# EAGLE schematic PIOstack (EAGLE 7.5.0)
COPYRIGHT: © 2015/2016 luani.de; LICENSE: CC-BY-SA 4.0; PROJEKT: PIOstack – Raspb. Pi Zero LAN, USB & Audio; REVISION: 1.1
Assembly variants: 2-Port Hub Minimal

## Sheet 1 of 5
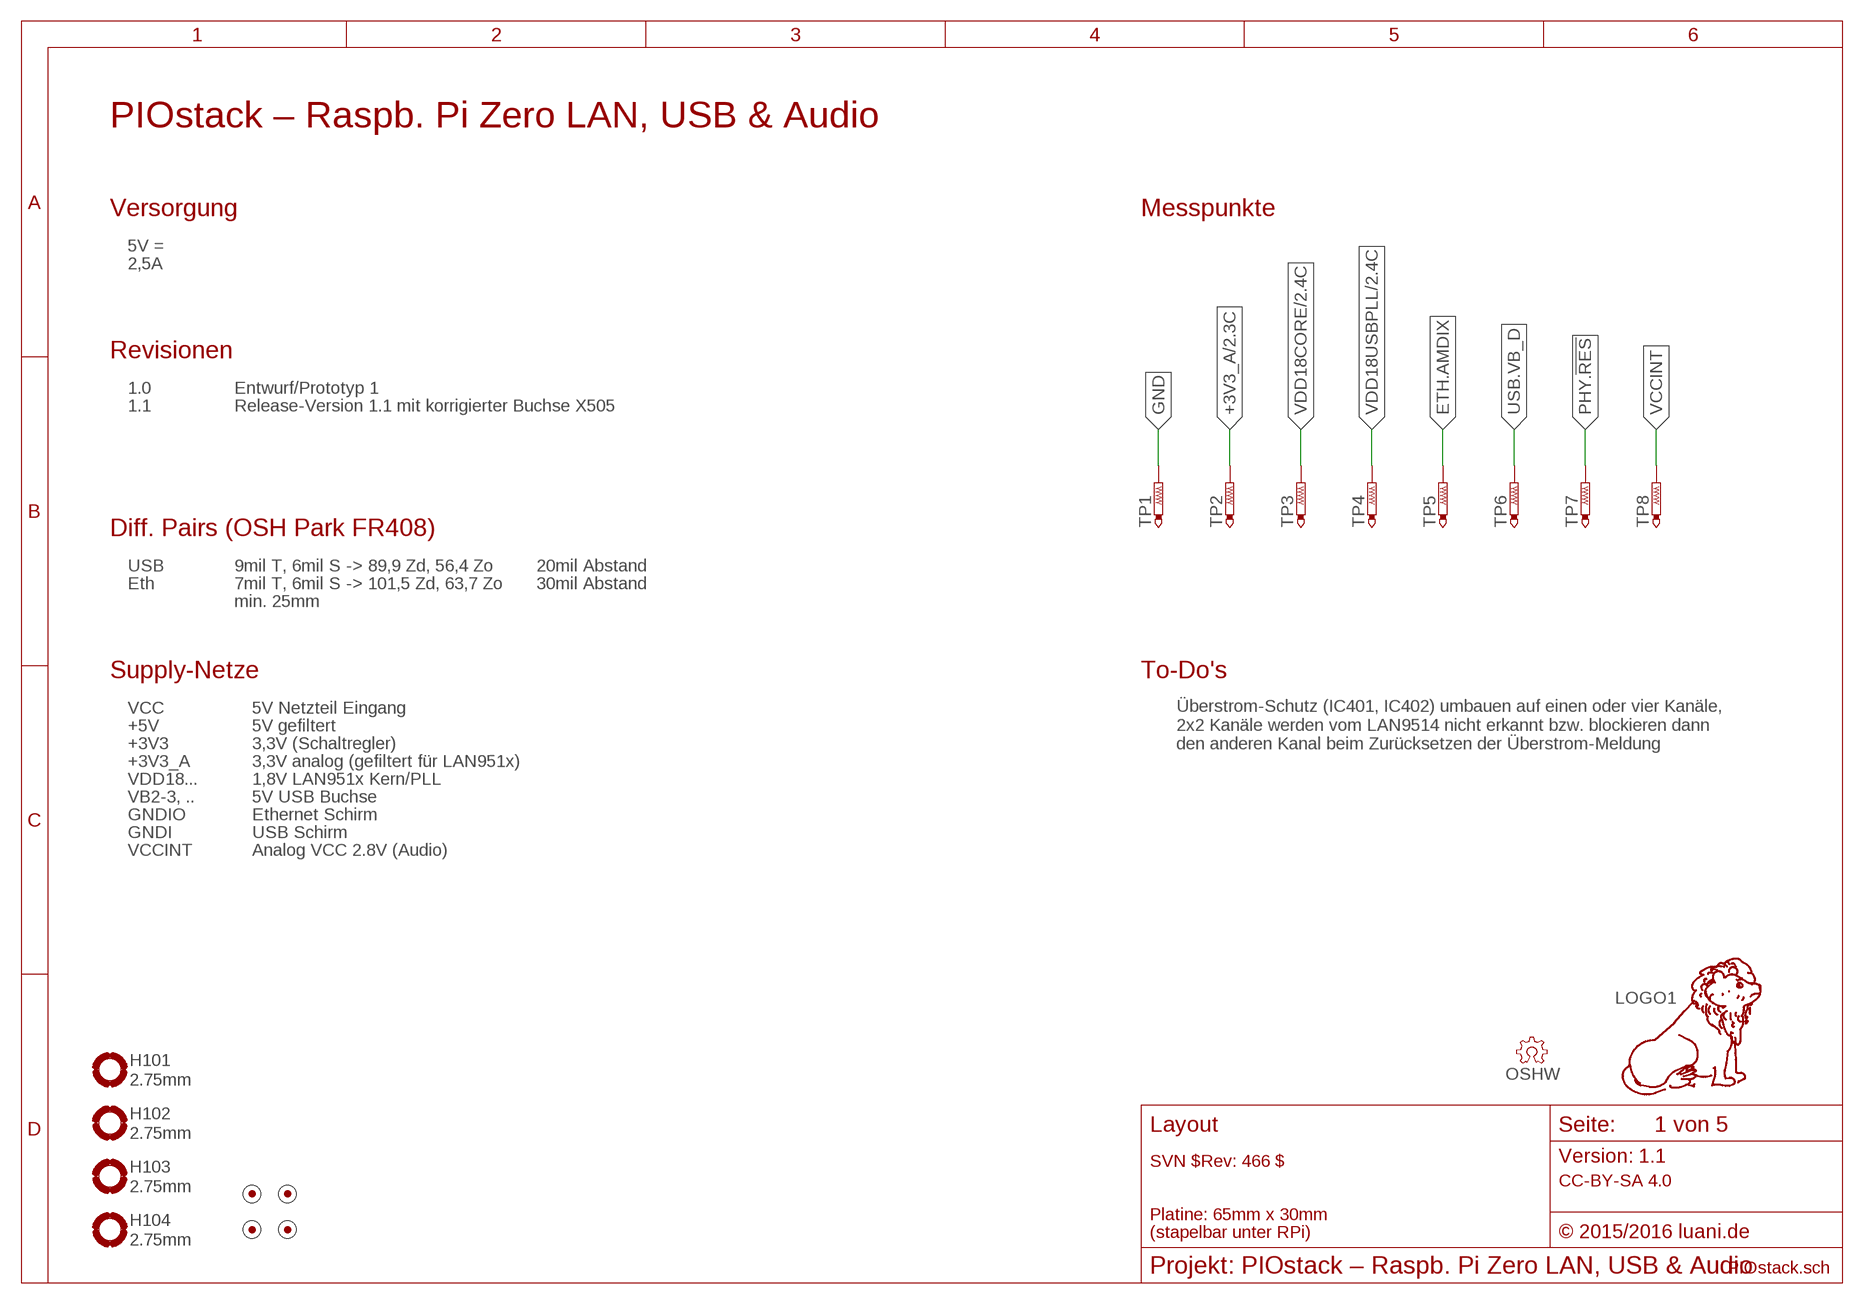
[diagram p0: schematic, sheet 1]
FRAME101 (FRAME_A4-L): TEXT-1: Layout; TEXT-2: SVN $Rev: 466 $; TEXT-4: Platine: 65mm x 30mm; TEXT-5: (stapelbar unter RPi)

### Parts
H101  2.75mm  HOLE_2.75R  [HOLE_2.75R]
H102  2.75mm  HOLE_2.75R  [HOLE_2.75R]
H103  2.75mm  HOLE_2.75R  [HOLE_2.75R]
H104  2.75mm  HOLE_2.75R  [HOLE_2.75R]
LOGO1  LOGO-10MM-TPLACE  [10MM-TPLACE]
MARK101  FIDUCIAL-1.0/CREAM  [FIDUCIAL-1MM/CREAM]
MARK102  FIDUCIAL-1.0/CREAM  [FIDUCIAL-1MM/CREAM]
MARK103  FIDUCIAL-1.0/CREAM  [FIDUCIAL-1MM/CREAM]
MARK104  FIDUCIAL-1.0/CREAM  [FIDUCIAL-1MM/CREAM]
OSHW  OSHW-3MM-FILL-TPLACE  [OSHW-FILL-3MM-TPLACE]
TP1  PTR1TP07R  [TP07R]
TP2  PTR1TP07R  [TP07R]
TP3  PTR1TP07R  [TP07R]
TP4  PTR1TP07R  [TP07R]
TP5  PTR1TP07R  [TP07R]
TP6  PTR1TP07R  [TP07R]
TP7  PTR1TP07R  [TP07R]
TP8  PTR1TP07R  [TP07R]

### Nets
+3V3_A: TP2.TP ; also sheet 2,3
ETH.AMDIX: TP5.TP ; also sheet 3
GND: TP1.TP ; also sheet 2,3,4,5
PHY.!RES: TP7.TP ; also sheet 2
USB.VB_D: TP6.TP ; also sheet 4
VCCINT: TP8.TP ; also sheet 5
VDD18CORE: TP3.TP ; also sheet 2
VDD18USBPLL: TP4.TP ; also sheet 2

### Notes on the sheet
- Versorgung | Messpunkte
- 5V =
- 2,5A
- Revisionen
- 1.0 | Entwurf/Prototyp 1
- 1.1 | Release-Version 1.1 mit korrigierter Buchse X505
- Diff. Pairs (OSH Park FR408)
- USB | 9mil T, 6mil S -> 89,9 Zd, 56,4 Zo | 20mil Abstand
- Eth | 7mil T, 6mil S -> 101,5 Zd, 63,7 Zo | 30mil Abstand
- min. 25mm
- Supply-Netze | To-Do's
- VCC | 5V Netzteil Eingang
- +5V | 5V gefiltert
- +3V3 | 3,3V (Schaltregler)
- Überstrom-Schutz (IC401, IC402) umbauen auf einen oder vier Kanäle,
  2x2 Kanäle werden vom LAN9514 nicht erkannt bzw. blockieren dann
  den anderen Kanal beim Zurücksetzen der Überstrom-Meldung
- +3V3_A | 3,3V analog (gefiltert für LAN951x)
- VDD18... | 1,8V LAN951x Kern/PLL
- VB2-3, .. | 5V USB Buchse
- GNDIO | Ethernet Schirm
- GNDI | USB Schirm
- VCCINT | Analog VCC 2.8V (Audio)

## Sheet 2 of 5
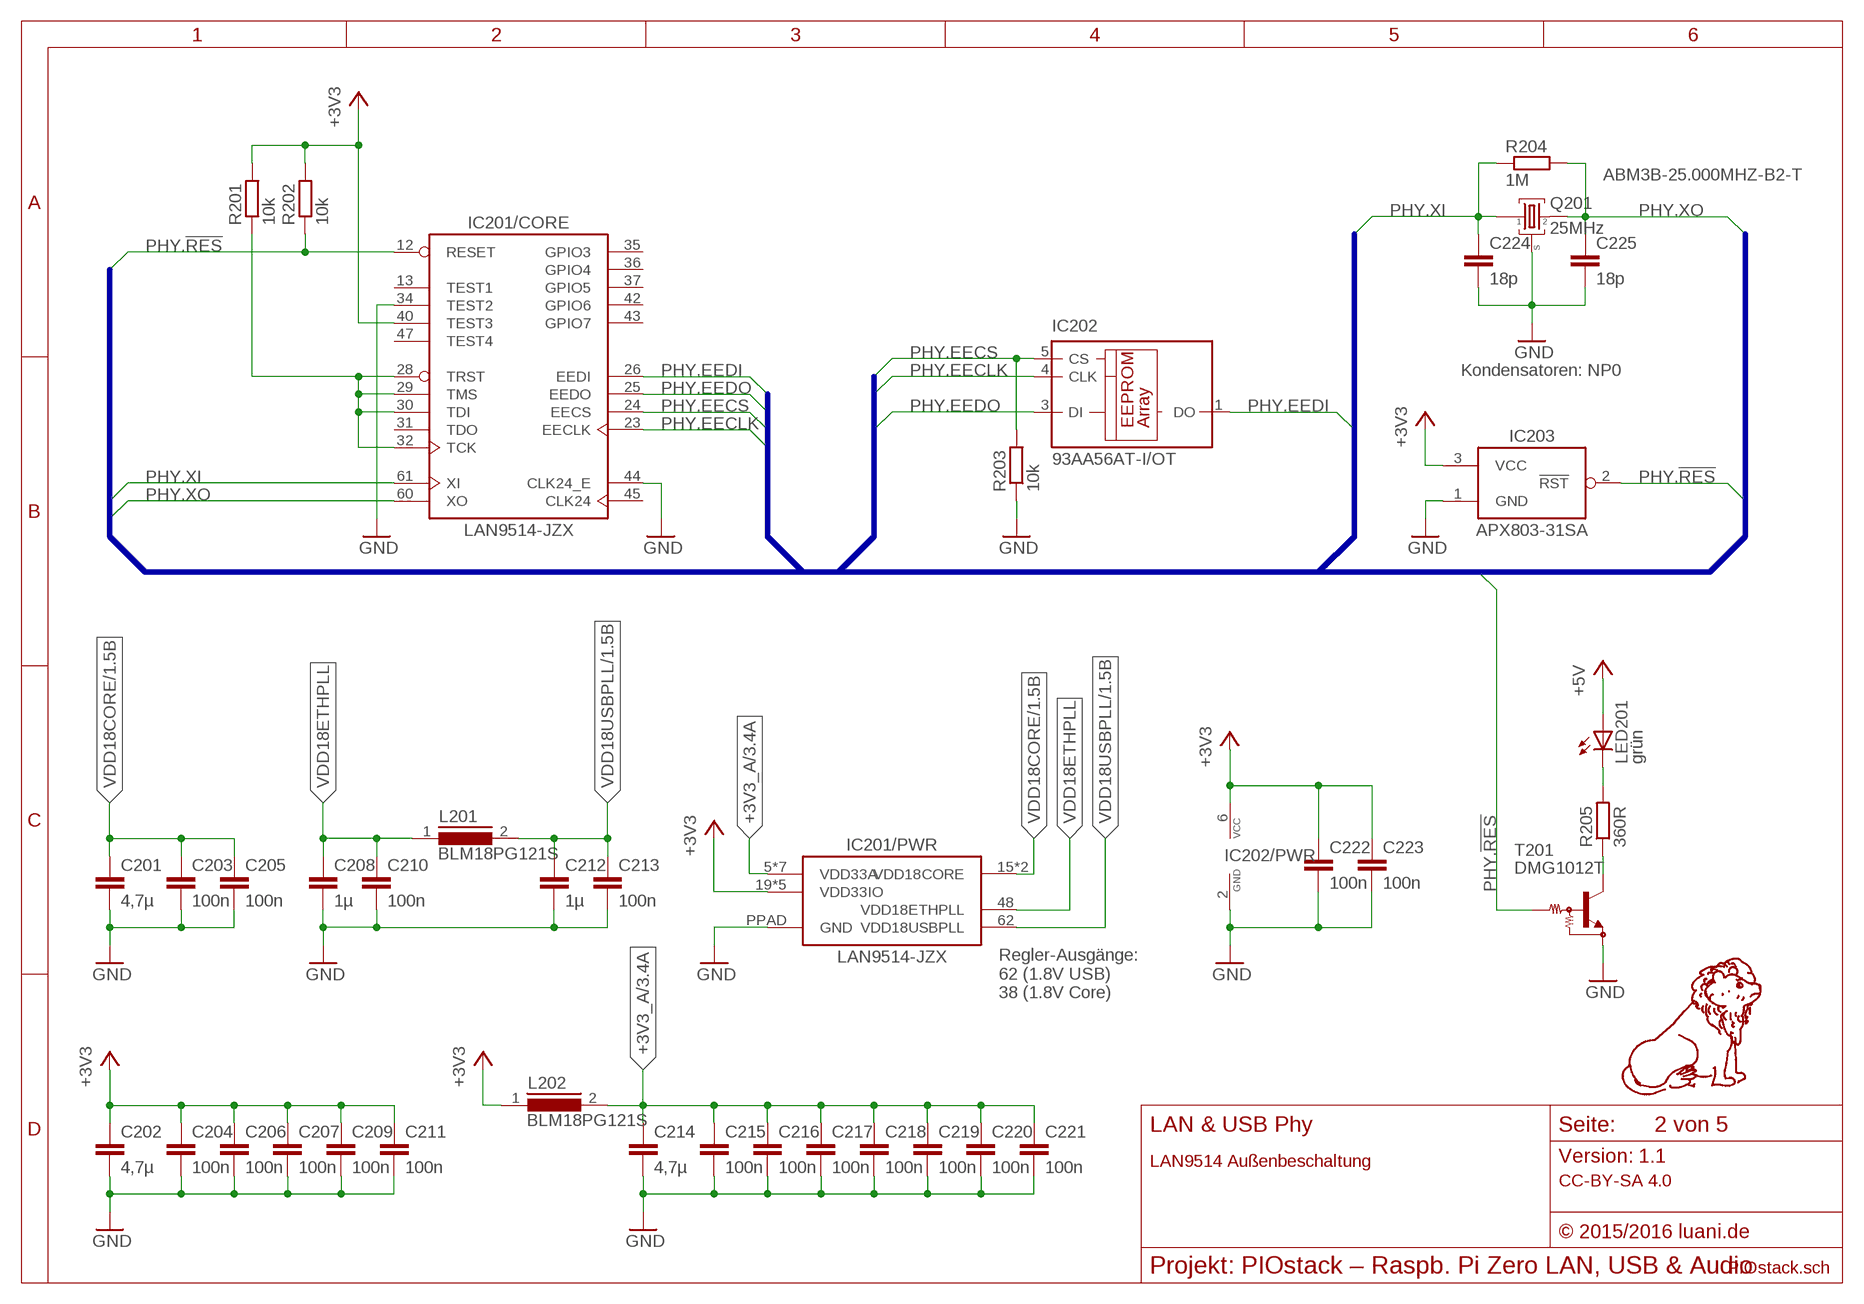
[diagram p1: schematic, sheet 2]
FRAME201 (FRAME_A4-L/LOGO): TEXT-1: LAN & USB Phy; TEXT-2: LAN9514 Außenbeschaltung

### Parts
C201  4,7µ  C-0603  [C-0603]
C202  4,7µ  C-0603  [C-0603]
C203  100n  C-0402  [C-0402]
C204  100n  C-0402  [C-0402]
C205  100n  C-0402  [C-0402]
C206  100n  C-0402  [C-0402]
C207  100n  C-0402  [C-0402]
C208  1µ  C-0603  [C-0603]
C209  100n  C-0402  [C-0402]
C210  100n  C-0402  [C-0402]
C211  100n  C-0402  [C-0402]
C212  1µ  C-0603  [C-0603]
C213  100n  C-0402  [C-0402]
C214  4,7µ  C-0603  [C-0603]
C215  100n  C-0402  [C-0402]
C216  100n  C-0402  [C-0402]
C217  100n  C-0402  [C-0402]
C218  100n  C-0402  [C-0402]
C219  100n  C-0402  [C-0402]
C220  100n  C-0402  [C-0402]
C221  100n  C-0402  [C-0402]
C222  100n  C-0402  [C-0402]  (not fitted in variant 2-Port Hub Minimal)
C223  100n  C-0402  [C-0402]  (not fitted in variant 2-Port Hub Minimal)
C224  18p  C-0402  [C-0402]
C225  18p  C-0402  [C-0402]
IC201  LAN9514-JZX  [QFN-64]
IC202  93AA56AT-I/OT  93LC46BT-I  [SOT23-6]  (not fitted in variant 2-Port Hub Minimal)
IC203  APX803-31SA  AP803_SA  [SOT-23/3]  (not fitted in variant 2-Port Hub Minimal)
L201  BLM18PG121S  INDUCTOR-BLM18  [BLM18P]
L202  BLM18PG121S  INDUCTOR-BLM18  [BLM18P]
LED201  grün  LED-CHIPLED-0603  [CHIPLED-0603]  (not fitted in variant 2-Port Hub Minimal)
Q201  25MHz  CRYSTAL-SHIELD_ABM3B  [ABRACON_ABM3B]
R201  10k  R-0402  [R-0402]
R202  10k  R-0402  [R-0402]
R203  10k  R-0402  [R-0402]  (not fitted in variant 2-Port Hub Minimal)
R204  1M  R-0402  [R-0402]
R205  360R  R-0402  [R-0402]  (not fitted in variant 2-Port Hub Minimal)
T201  DMG1012T  NPN-DIGITAL-DTC114  [SC75]  (not fitted in variant 2-Port Hub Minimal)

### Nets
+3V3: C202.1 C204.1 C206.1 C207.1 C209.1 C211.1 C222.1 C223.1 IC201.19(/PWR:VDD33IO) IC201.27(/PWR:VDD33IO) IC201.33(/PWR:VDD33IO) IC201.39(/PWR:VDD33IO) IC201.40(/CORE:TEST3) IC201.46(/PWR:VDD33IO) IC202.6(VCC) IC203.3(VCC) L202.1 R201.2 R202.2 ; also sheet 3,4,5
+3V3_A: C214.1 C215.1 C216.1 C217.1 C218.1 C219.1 C220.1 C221.1 IC201.5(/PWR:VDD33A) IC201.10(/PWR:VDD33A) IC201.49(/PWR:VDD33A) IC201.51(/PWR:VDD33A) IC201.54(/PWR:VDD33A) IC201.57(/PWR:VDD33A) IC201.64(/PWR:VDD33A) L202.2 ; also sheet 1,3
+5V: LED201.A ; also sheet 4,5
GND: C201.2 C202.2 C203.2 C204.2 C205.2 C206.2 C207.2 C208.2 C209.2 C210.2 C211.2 C212.2 C213.2 C214.2 C215.2 C216.2 C217.2 C218.2 C219.2 C220.2 C221.2 C222.2 C223.2 C224.2 C225.2 IC201.34(/CORE:TEST2) IC201.44(/CORE:CLK24_E) IC201.PPAD(/PWR:GND) IC202.2(GND) IC203.1(GND) Q201.S@0(S) Q201.S@1(S) R203.1 T201.2(E) ; also sheet 1,3,4,5
N$6: LED201.C R205.2
N$7: R205.1 T201.3(C)
PHY.!RES: IC201.12(/CORE:RESET) IC203.2(!RST) R202.1 T201.1(B) ; also sheet 1
PHY.EECLK: IC201.23(/CORE:EECLK) IC202.4(CLK)
PHY.EECS: IC201.24(/CORE:EECS) IC202.5(CS) R203.2
PHY.EEDI: IC201.26(/CORE:EEDI) IC202.1(DO)
PHY.EEDO: IC201.25(/CORE:EEDO) IC202.3(DI)
PHY.JTAG-PU: IC201.28(/CORE:TRST) IC201.29(/CORE:TMS) IC201.30(/CORE:TDI) IC201.32(/CORE:TCK) R201.1
PHY.XI [Takt]: C224.1 IC201.61(/CORE:XI) Q201.1 R204.1
PHY.XO [Takt]: C225.1 IC201.60(/CORE:XO) Q201.2 R204.2
VDD18CORE: C201.1 C203.1 C205.1 IC201.15(/PWR:VDD18CORE) IC201.38(/PWR:VDD18CORE) ; also sheet 1
VDD18ETHPLL: C208.1 C210.1 IC201.48(/PWR:VDD18ETHPLL) L201.1
VDD18USBPLL: C212.1 C213.1 IC201.62(/PWR:VDD18USBPLL) L201.2 ; also sheet 1
Unconnected: IC201.13(/CORE:TEST1) IC201.31(/CORE:TDO) IC201.35(/CORE:GPIO3) IC201.36(/CORE:GPIO4) IC201.37(/CORE:GPIO5) IC201.42(/CORE:GPIO6) IC201.43(/CORE:GPIO7) IC201.45(/CORE:CLK24) IC201.47(/CORE:TEST4)

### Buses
PHY:PHY.EEDI,PHY.EEDO,PHY.EECS,PHY.EECLK,PHY.!RES,PHY.XI,PHY.XO

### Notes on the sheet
- Kondensatoren: NP0
- Regler-Ausgänge:
  62 (1.8V USB)
  38 (1.8V Core)

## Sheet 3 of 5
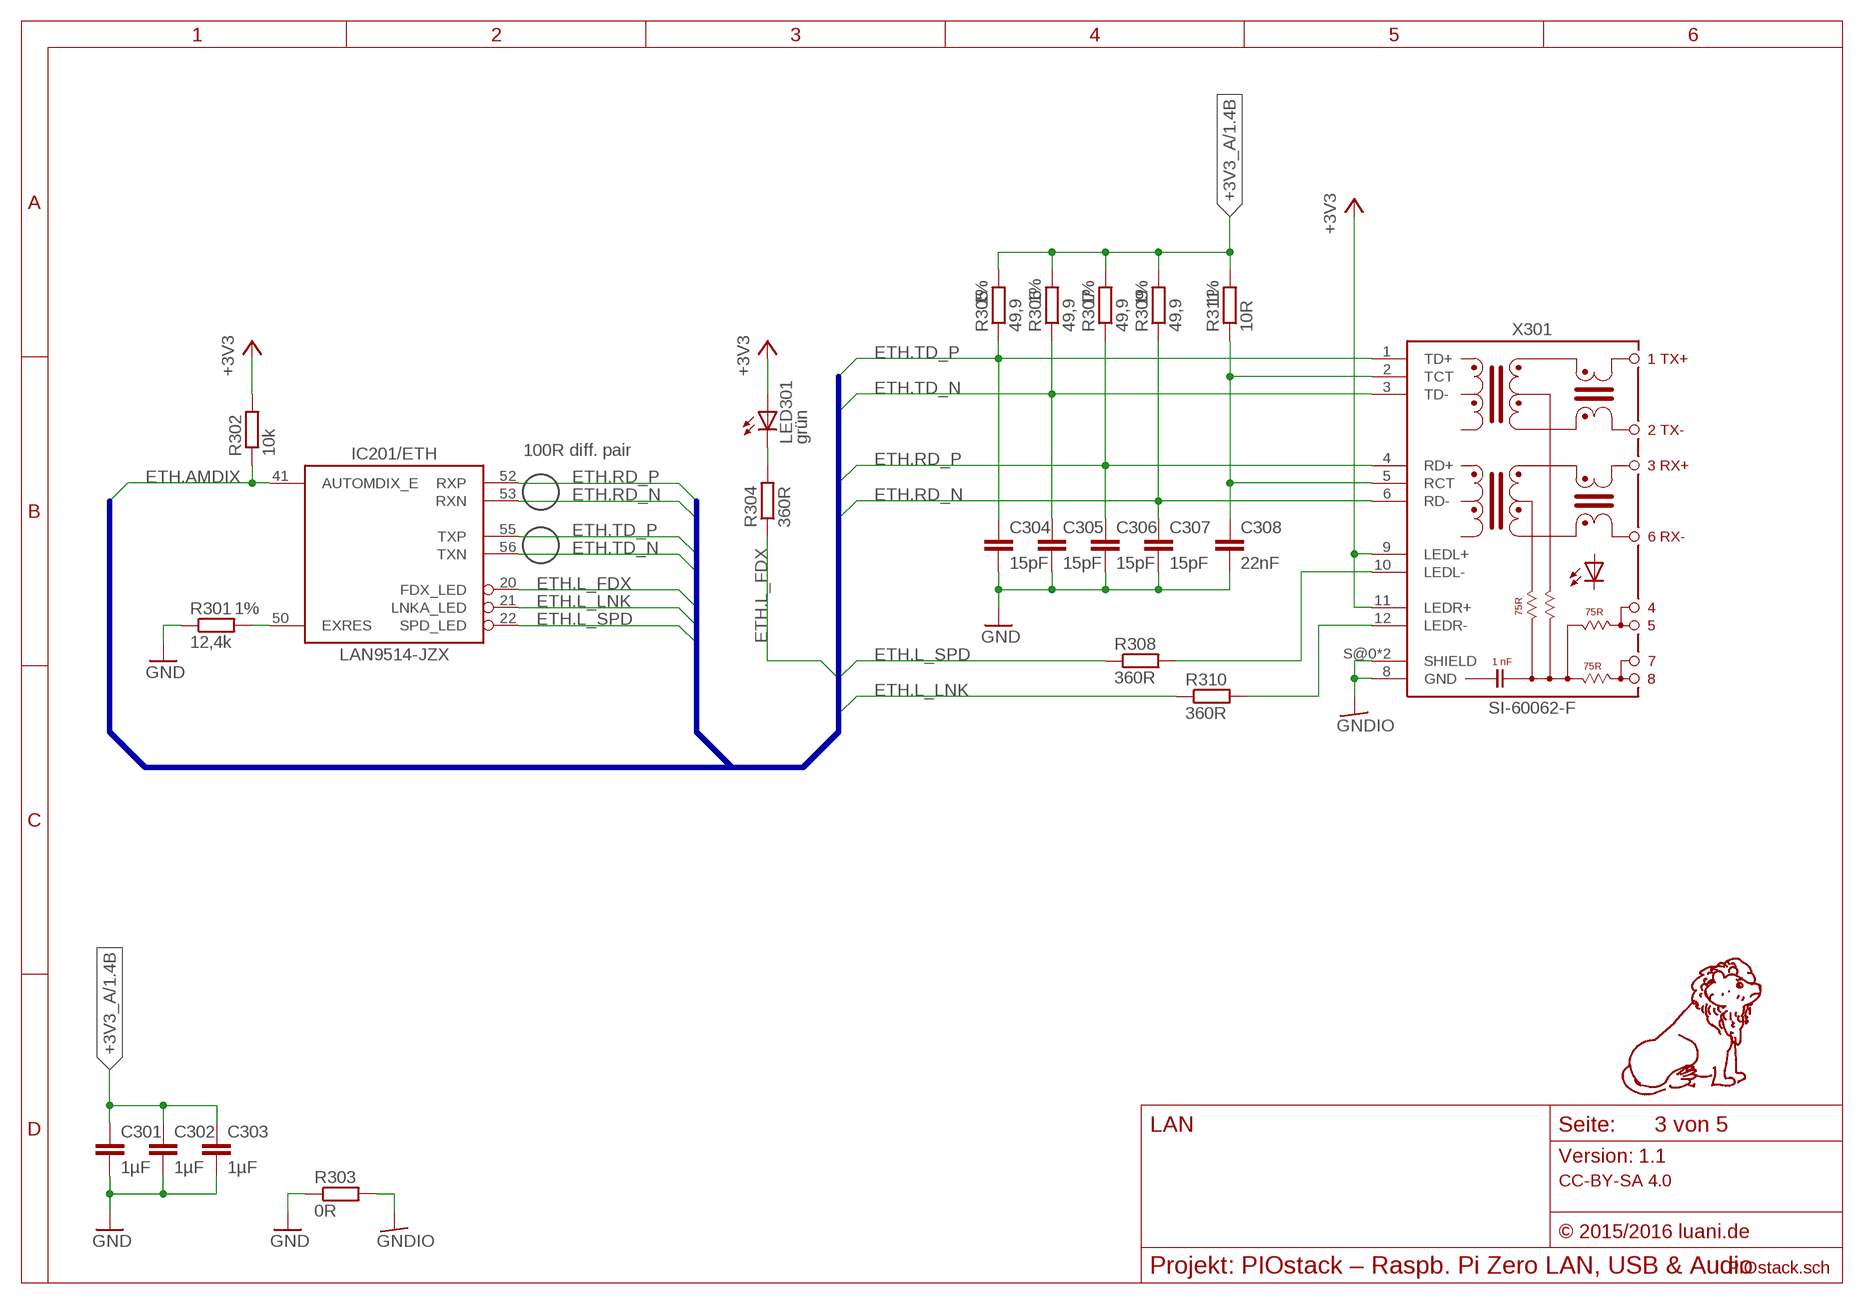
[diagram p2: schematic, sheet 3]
FRAME301 (FRAME_A4-L/LOGO): TEXT-1: LAN

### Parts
C301  1µF  C-0603  [C-0603]
C302  1µF  C-0603  [C-0603]
C303  1µF  C-0603  [C-0603]
C304  15pF  C-0402  [C-0402]
C305  15pF  C-0402  [C-0402]
C306  15pF  C-0402  [C-0402]
C307  15pF  C-0402  [C-0402]
C308  22nF  C-0603  [C-0603]
LED301  grün  LED-CHIPLED-0603  [CHIPLED-0603]  (not fitted in variant 2-Port Hub Minimal)
R301  12,4k  R-0603  [R-0603]
R302  10k  R-0402  [R-0402]
R303  0R  R-0805  [R-0805]
R304  360R  R-0402  [R-0402]  (not fitted in variant 2-Port Hub Minimal)
R305  49,9  R-0402  [R-0402]
R306  49,9  R-0402  [R-0402]
R307  49,9  R-0402  [R-0402]
R308  360R  R-0402  [R-0402]
R309  49,9  R-0402  [R-0402]
R310  360R  R-0402  [R-0402]
R311  10R  R-0603  [R-0603]
X301  SI-60062-F  MAGJACK-LED_SI-60062-F  [BEL_SI-60062-F]

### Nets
+3V3: LED301.A R302.2 X301.9(LEDL+) X301.11(LEDR+) ; also sheet 2,4,5
+3V3_A: C301.1 C302.1 C303.1 R305.2 R306.2 R307.2 R309.2 R311.2 ; also sheet 1,2
ETH.AMDIX: IC201.41(/ETH:AUTOMDIX_E) R302.1 ; also sheet 1
ETH.L_FDX: IC201.20(/ETH:FDX_LED) R304.1
ETH.L_LNK: IC201.21(/ETH:LNKA_LED) R310.1
ETH.L_SPD: IC201.22(/ETH:SPD_LED) R308.1
ETH.RD_N [Ethernet-Diffpair]: C307.1 IC201.53(/ETH:RXN) R309.1 X301.6(RD-)
ETH.RD_P [Ethernet-Diffpair]: C306.1 IC201.52(/ETH:RXP) R307.1 X301.4(RD+)
ETH.TD_N [Ethernet-Diffpair]: C305.1 IC201.56(/ETH:TXN) R306.1 X301.3(TD-)
ETH.TD_P [Ethernet-Diffpair]: C304.1 IC201.55(/ETH:TXP) R305.1 X301.1(TD+)
ETH.TR-CT: C308.1 R311.1 X301.2(TCT) X301.5(RCT)
GND: C301.2 C302.2 C303.2 C304.2 C305.2 C306.2 C307.2 C308.2 R301.1 R303.1 ; also sheet 1,2,4,5
GNDIO [Schirm]: R303.2 X301.8(GND) X301.S@0(SHIELD) X301.S@1(SHIELD)
N$1: R308.2 X301.10(LEDL-)
N$2: IC201.50(/ETH:EXRES) R301.2
N$12: R310.2 X301.12(LEDR-)
N$14: LED301.C R304.2

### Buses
ETH.TD_P,ETH.TD_N,ETH.RD_P,ETH.RD_N,ETH.AMDIX,ETH.L_FDX,ETH.L_LNK,ETH.L_SPD

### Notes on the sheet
- 100R diff. pair

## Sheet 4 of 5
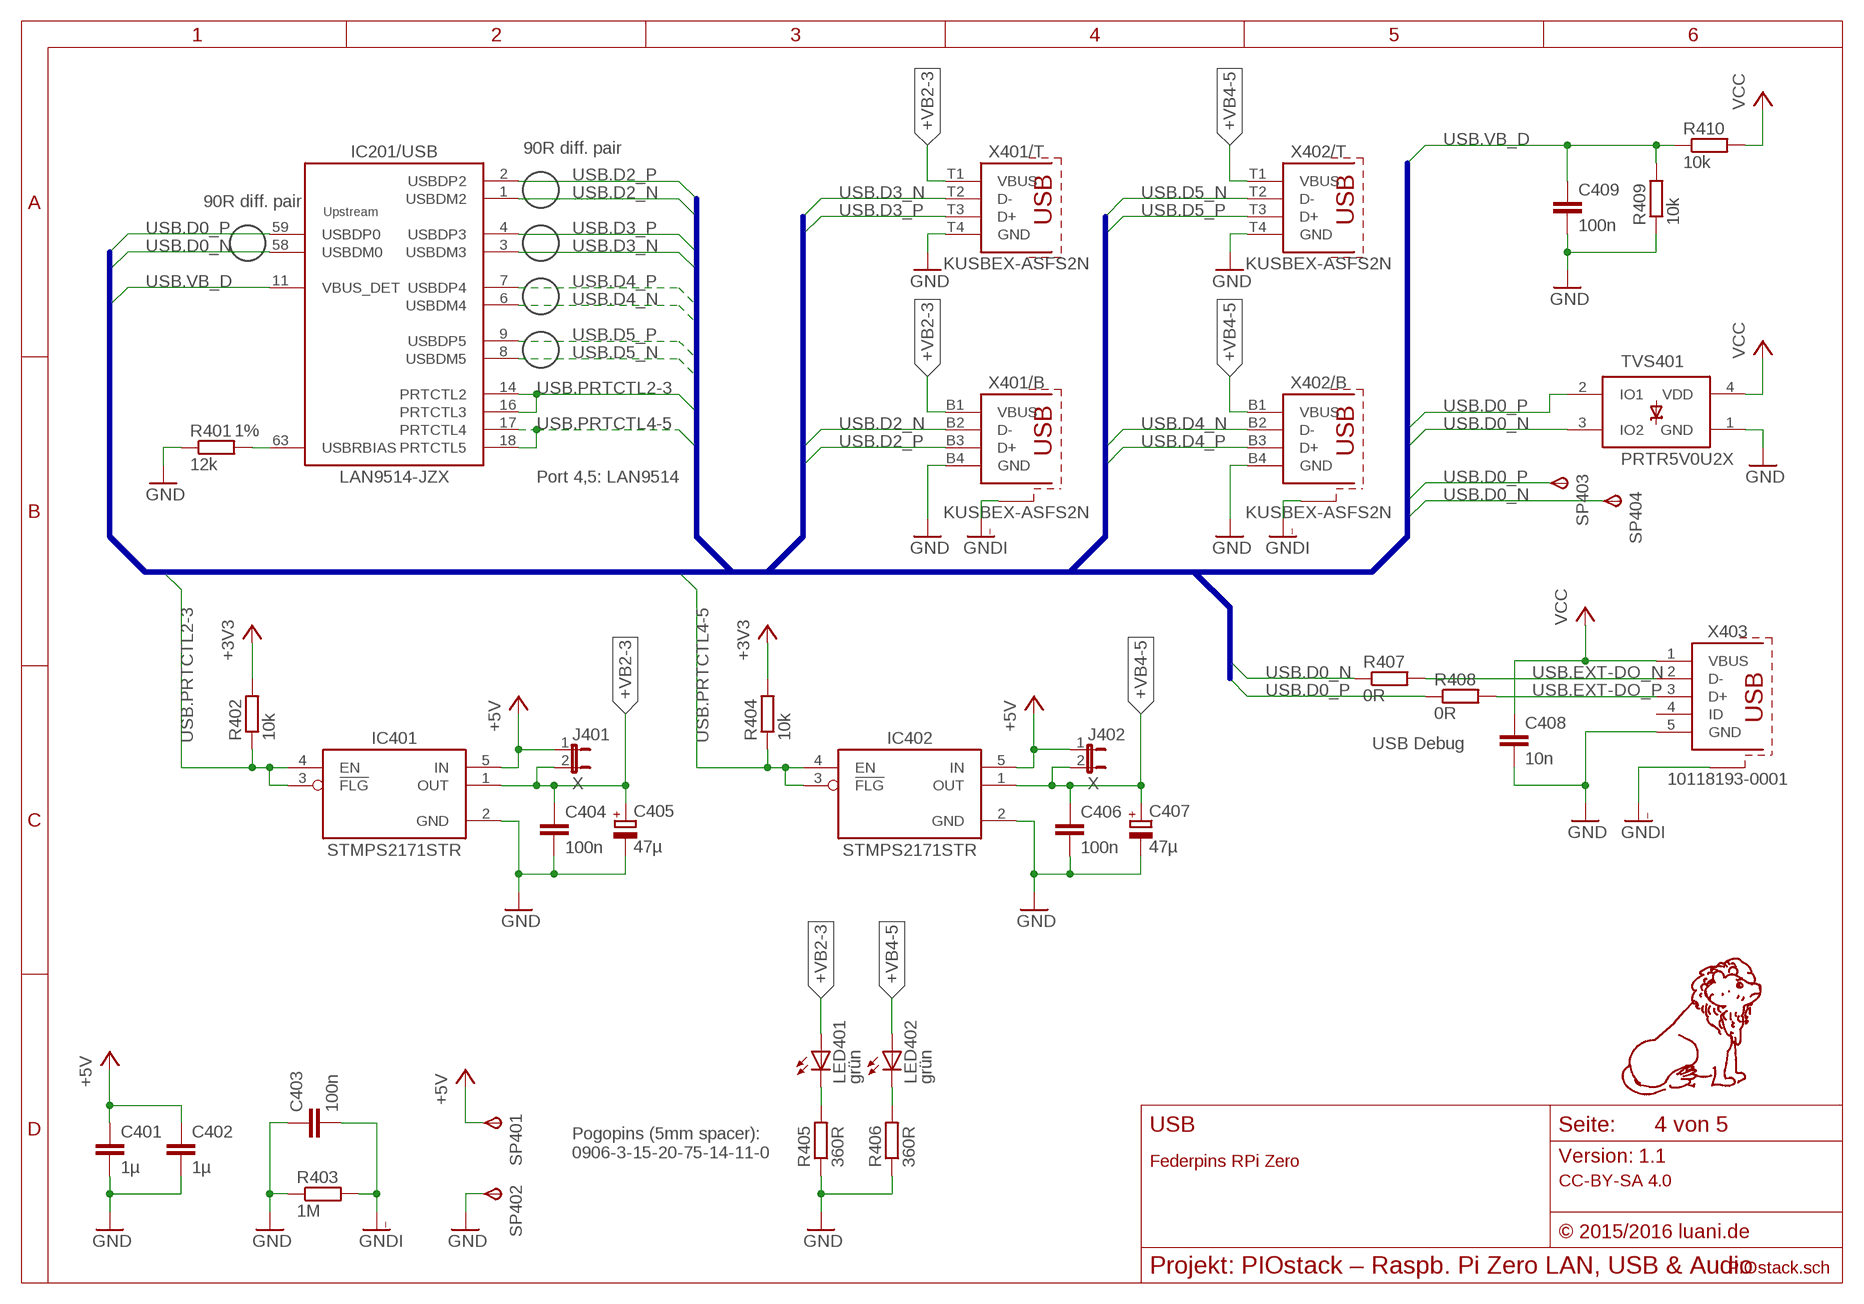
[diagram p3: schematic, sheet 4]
FRAME401 (FRAME_A4-L/LOGO): TEXT-1: USB; TEXT-2: Federpins RPi Zero

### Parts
C401  1µ  C-0603  [C-0603]  (not fitted in variant 2-Port Hub Minimal)
C402  1µ  C-0603  [C-0603]  (not fitted in variant 2-Port Hub Minimal)
C403  100n  C-0805  [C-0805]
C404  100n  C-0805  [C-0805]  (not fitted in variant 2-Port Hub Minimal)
C405  47µ  CPOL-EUE2-5  [E2-5]  (not fitted in variant 2-Port Hub Minimal)
C406  100n  C-0805  [C-0805]  (not fitted in variant 2-Port Hub Minimal)
C407  47µ  CPOL-EUE2-5  [E2-5]  (not fitted in variant 2-Port Hub Minimal)
C408  10n  C-0603  [C-0603]
C409  100n  C-0402  [C-0402]
IC401  STMPS2171STR  AP2161_AW  [SOT-23/5]  (not fitted in variant 2-Port Hub Minimal)
IC402  STMPS2171STR  AP2161_AW  [SOT-23/5]
J401  X  JUMPER-2-R  [JUMPER-2-R]
J402  X  JUMPER-2-R  [JUMPER-2-R]  (not fitted in variant 2-Port Hub Minimal)
LED401  grün  LED-CHIPLED-0603  [CHIPLED-0603]  (not fitted in variant 2-Port Hub Minimal)
LED402  grün  LED-CHIPLED-0603  [CHIPLED-0603]  (not fitted in variant 2-Port Hub Minimal)
R401  12k  R-0603  [R-0603]
R402  10k  R-0402  [R-0402]  (not fitted in variant 2-Port Hub Minimal)
R403  1M  R-0805  [R-0805]
R404  10k  R-0402  [R-0402]  (not fitted in variant 2-Port Hub Minimal)
R405  360R  R-0402  [R-0402]  (not fitted in variant 2-Port Hub Minimal)
R406  360R  R-0402  [R-0402]  (not fitted in variant 2-Port Hub Minimal)
R407  0R  R-0402  [R-0402]  (not fitted in variant 2-Port Hub Minimal)
R408  0R  R-0402  [R-0402]  (not fitted in variant 2-Port Hub Minimal)
R409  10k  R-0402  [R-0402]
R410  10k  R-0402  [R-0402]
SP401  TESTPOINT-0906  [TESTPOINT-0906]
SP402  TESTPOINT-0906  [TESTPOINT-0906]
SP403  TESTPOINT-0906  [TESTPOINT-0906]
SP404  TESTPOINT-0906  [TESTPOINT-0906]
TVS401  PRTR5V0U2X  2-ARRAY-NXP-PRTR  [SOT143B]
X401  KUSBEX-ASFS2N  USB-4-D_KUSBEX-ASFS2N  [KYCON_KUSBEX-ASFS2N]
X402  KUSBEX-ASFS2N  USB-4-D_KUSBEX-ASFS2N  [KYCON_KUSBEX-ASFS2N]  (not fitted in variant 2-Port Hub Minimal)
X403  10118193-0001  USB-5_10118193-0001  [FCI_10118193]

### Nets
+3V3: R402.2 R404.2 ; also sheet 2,3,5
+5V: C401.1 C402.1 IC401.5(IN) IC402.5(IN) J401.1 J402.1 SP401.TP(PP) ; also sheet 2,5
+VB2-3: C404.1 C405.+ IC401.1(OUT) J401.2 LED401.A X401.B1(/B:VBUS) X401.T1(/T:VBUS)
+VB4-5: C406.1 C407.+ IC402.1(OUT) J402.2 LED402.A X402.B1(/B:VBUS) X402.T1(/T:VBUS)
GND: C401.2 C402.2 C403.1 C404.2 C405.- C406.2 C407.- C408.2 C409.2 IC401.2(GND) IC402.2(GND) R401.1 R403.1 R405.1 R406.1 R409.1 SP402.TP(PP) TVS401.1(GND) X401.B4(/B:GND) X401.T4(/T:GND) X402.B4(/B:GND) X402.T4(/T:GND) X403.5(GND) ; also sheet 1,2,3,5
GNDI [Schirm]: C403.2 R403.2 X401.S@0(/B:SHIELD) X401.S@1(/B:SHIELD) X401.S@2(/B:SHIELD) X401.S@3(/B:SHIELD) X402.S@0(/B:SHIELD) X402.S@1(/B:SHIELD) X402.S@2(/B:SHIELD) X402.S@3(/B:SHIELD) X403.S@0(SHIELD) X403.S@1(SHIELD) X403.S@2(SHIELD) X403.S@3(SHIELD) X403.S@4(SHIELD) X403.S@5(SHIELD)
N$3: IC201.63(/USB:USBRBIAS) R401.2
N$10: LED402.C R406.2
N$13: LED401.C R405.2
USB.D0_N [USB-Diffpair]: IC201.58(/USB:USBDM0) R407.1 SP404.TP(PP) TVS401.3(IO2)
USB.D0_P [USB-Diffpair]: IC201.59(/USB:USBDP0) R408.1 SP403.TP(PP) TVS401.2(IO1)
USB.D2_N [USB-Diffpair]: IC201.1(/USB:USBDM2) X401.B2(/B:D-)
USB.D2_P [USB-Diffpair]: IC201.2(/USB:USBDP2) X401.B3(/B:D+)
USB.D3_N [USB-Diffpair]: IC201.3(/USB:USBDM3) X401.T2(/T:D-)
USB.D3_P [USB-Diffpair]: IC201.4(/USB:USBDP3) X401.T3(/T:D+)
USB.D4_N [USB-Diffpair]: IC201.6(/USB:USBDM4) X402.B2(/B:D-)
USB.D4_P [USB-Diffpair]: IC201.7(/USB:USBDP4) X402.B3(/B:D+)
USB.D5_N [USB-Diffpair]: IC201.8(/USB:USBDM5) X402.T2(/T:D-)
USB.D5_P [USB-Diffpair]: IC201.9(/USB:USBDP5) X402.T3(/T:D+)
USB.EXT-DO_N [USB-Diffpair]: R407.2 X403.2(D-)
USB.EXT-DO_P [USB-Diffpair]: R408.2 X403.3(D+)
USB.PRTCTL2-3: IC201.14(/USB:PRTCTL2) IC201.16(/USB:PRTCTL3) IC401.3(!FLG) IC401.4(EN) R402.1
USB.PRTCTL4-5: IC201.17(/USB:PRTCTL4) IC201.18(/USB:PRTCTL5) IC402.3(!FLG) IC402.4(EN) R404.1
USB.VB_D: C409.1 IC201.11(/USB:VBUS_DET) R409.2 R410.1 ; also sheet 1
VCC [Standardleiter neben Diffpair]: C408.1 R410.2 TVS401.4(VDD) X403.1(VBUS) ; also sheet 5
Unconnected: X403.4(ID)

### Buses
USB:USB.D0_P,USB.D0_N,USB.D2_P,USB.D2_N,USB.D3_P,USB.D3_N,USB.D4_P,USB.D4_N,USB.D5_P,USB.D5_N,USB.PRTCTL2-3,USB.PRTCTL4-5,USB.VB_D

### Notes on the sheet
- 90R diff. pair
- 90R diff. pair
- Port 4,5: LAN9514
- USB Debug
- Pogopins (5mm spacer):
  0906-3-15-20-75-14-11-0

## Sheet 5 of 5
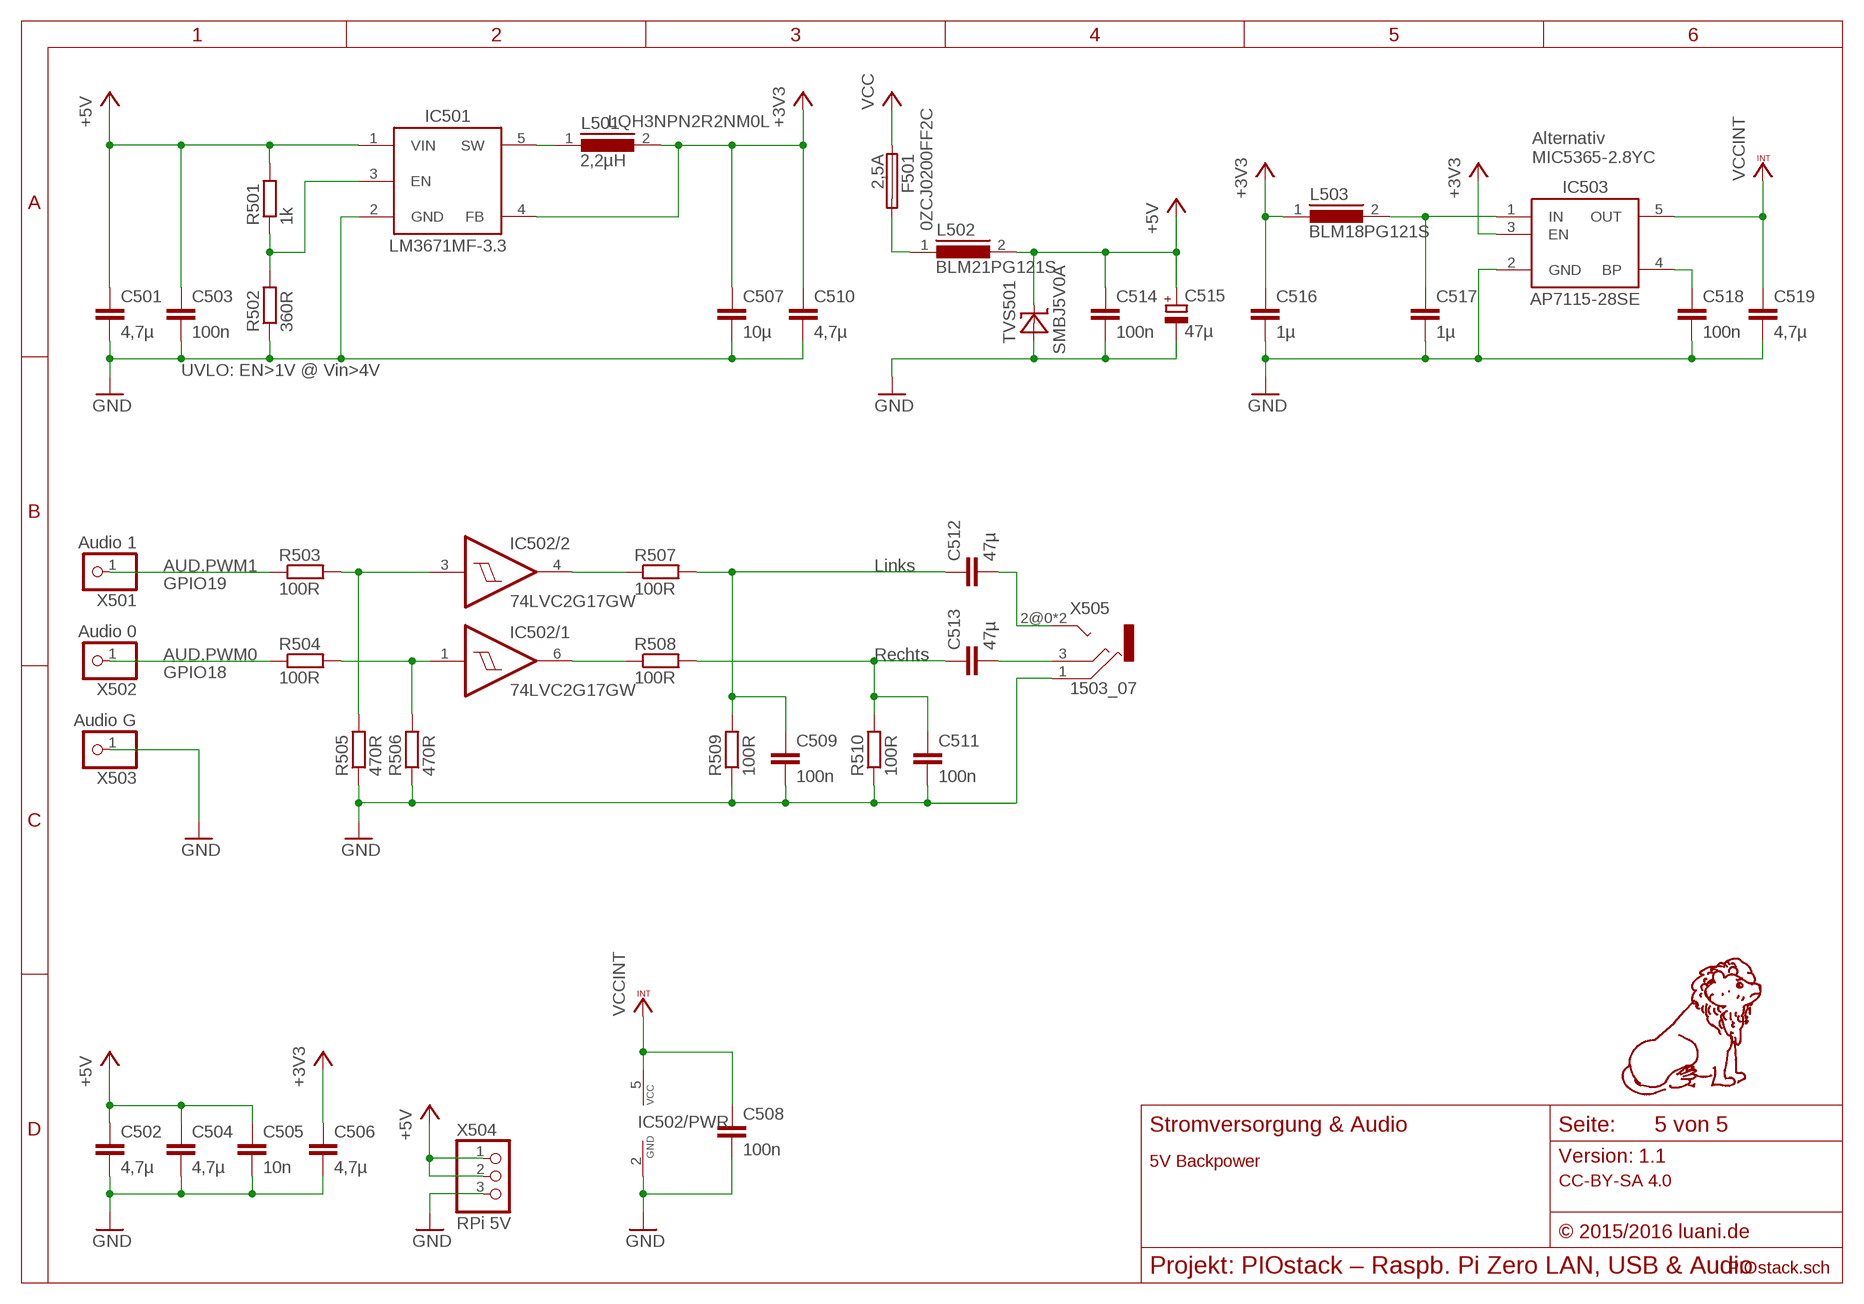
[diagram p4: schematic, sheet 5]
FRAME501 (FRAME_A4-L/LOGO): TEXT-1: Stromversorgung & Audio; TEXT-2: 5V Backpower

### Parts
C501  4,7µ  C-0805  [C-0805]
C502  4,7µ  C-0805  [C-0805]
C503  100n  C-0402  [C-0402]
C504  4,7µ  C-0805  [C-0805]
C505  10n  C-0603  [C-0603]
C506  4,7µ  C-0603  [C-0603]
C507  10µ  C-0805  [C-0805]
C508  100n  C-0402  [C-0402]  (not fitted in variant 2-Port Hub Minimal)
C509  100n  C-0402  [C-0402]  (not fitted in variant 2-Port Hub Minimal)
C510  4,7µ  C-0603  [C-0603]
C511  100n  C-0402  [C-0402]  (not fitted in variant 2-Port Hub Minimal)
C512  47µ  C-0805  [C-0805]  (not fitted in variant 2-Port Hub Minimal)
C513  47µ  C-0805  [C-0805]  (not fitted in variant 2-Port Hub Minimal)
C514  100n  C-0805  [C-0805]
C515  47µ  CPOL-EUE2-5  [E2-5]
C516  1µ  C-0603  [C-0603]  (not fitted in variant 2-Port Hub Minimal)
C517  1µ  C-0603  [C-0603]  (not fitted in variant 2-Port Hub Minimal)
C518  100n  C-0402  [C-0402]  (not fitted in variant 2-Port Hub Minimal)
C519  4,7µ  C-0603  [C-0603]  (not fitted in variant 2-Port Hub Minimal)
F501  2,5A  SMD-FUSE-1206  [BEL-1206]
IC501  LM3671MF-3.3  LM3671_MF  [SOT-23/5]
IC502  74LVC2G17GW  74LVC2G17_GW  [SOT-363/6]  (not fitted in variant 2-Port Hub Minimal)
IC503  AP7115-28SE  AP7115_SE  [SOT-353/5]  (not fitted in variant 2-Port Hub Minimal)
L501  2,2µH  L_LQH3NP  [MURATA_LQH3NP]
L502  BLM21PG121S  INDUCTOR-BLM21  [BLM21P]
L503  BLM18PG121S  INDUCTOR-BLM18  [BLM18P]  (not fitted in variant 2-Port Hub Minimal)
R501  1k  R-0402  [R-0402]
R502  360R  R-0402  [R-0402]
R503  100R  R-0402  [R-0402]  (not fitted in variant 2-Port Hub Minimal)
R504  100R  R-0402  [R-0402]  (not fitted in variant 2-Port Hub Minimal)
R505  470R  R-0402  [R-0402]  (not fitted in variant 2-Port Hub Minimal)
R506  470R  R-0402  [R-0402]  (not fitted in variant 2-Port Hub Minimal)
R507  100R  R-0402  [R-0402]  (not fitted in variant 2-Port Hub Minimal)
R508  100R  R-0402  [R-0402]  (not fitted in variant 2-Port Hub Minimal)
R509  100R  R-0402  [R-0402]  (not fitted in variant 2-Port Hub Minimal)
R510  100R  R-0402  [R-0402]  (not fitted in variant 2-Port Hub Minimal)
TVS501  SMBJ5V0A  TVS-UNI-SM6T-X-A  [DO214-AA]
X501  Audio 1  PINHD-1X1  [1X01]  (not fitted in variant 2-Port Hub Minimal)
X502  Audio 0  PINHD-1X1  [1X01]  (not fitted in variant 2-Port Hub Minimal)
X503  Audio G  PINHD-1X1  [1X01]  (not fitted in variant 2-Port Hub Minimal)
X504  RPi 5V  PINHD-1X3  [1X03]
X505  1503_07  STEREO-JACK_1503-07  [LUMBERG_1503-07]  (not fitted in variant 2-Port Hub Minimal)

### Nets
+3V3: C506.1 C507.1 C510.1 C516.1 IC501.4(FB) IC503.3(EN) L501.2 L503.1 ; also sheet 2,3,4
+5V: C501.1 C502.1 C503.1 C504.1 C505.1 C514.1 C515.+ IC501.1(VIN) L502.2 R501.2 TVS501.K X504.1 X504.2 ; also sheet 2,4
AUD.PWM0: R504.1 X502.1
AUD.PWM1: R503.1 X501.1
GND: C501.2 C502.2 C503.2 C504.2 C505.2 C506.2 C507.2 C508.2 C509.2 C510.2 C511.2 C514.2 C515.- C516.2 C517.2 C518.2 C519.2 IC501.2(GND) IC502.2(/PWR:GND) IC503.2(GND) R502.1 R505.1 R506.1 R509.1 R510.1 TVS501.A X503.1 X504.3 X505.1(E) ; also sheet 1,2,3,4
IC501.SW: IC501.5(SW) L501.1
IC503.BP: C518.1 IC503.4(BP)
IC503.VIN: C517.1 IC503.1(IN) L503.2
N$4: IC501.3(EN) R501.1 R502.2
N$9: C509.1 C512.1 R507.2 R509.2
N$11: F501.2 L502.1
N$15: C511.1 C513.1 R508.2 R510.2
N$16: C512.2 X505.2@0(T) X505.2@1(T)
N$17: C513.2 X505.3(R)
N$18: IC502.4(/2:O) R507.1
N$19: IC502.6(/1:O) R508.1
N$20: IC502.3(/2:I) R503.2 R505.2
N$21: IC502.1(/1:I) R504.2 R506.2
VCC [Standardleiter neben Diffpair]: F501.1 ; also sheet 4
VCCINT: C508.1 C519.1 IC502.5(/PWR:VCC) IC503.5(OUT) ; also sheet 1

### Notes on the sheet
- Alternativ
  MIC5365-2.8YC
- UVLO: EN>1V @ Vin>4V
- Links
- GPIO19
- Rechts
- GPIO18

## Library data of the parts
C201-C225 C301-C308 C501 C502 C504-C507 C510 C512-C514 C516 C517 C519 = leo_rc-smd:C: Capacitor
C401-C404 C406 C408 C409 C503 C508 C509 C511 C518 = luani_rc-smd:C: Capacitor
C405 C407 C515 = rcl:CPOL-EU: POLARIZED CAPACITOR, European symbol
F501 = leo_fuse-smd:SMD-FUSE: Surface Mount Fuses; ARTIKEL: 0ZCJ0200FF2C
H101-H104 = luani_mounting:HOLE: Mounting holes
IC201 = luani_chips:LAN9514: LAN9514 4 Port USB Hub 1 Port 10/100 LAN
IC202 = leo_chip-memory:93LC46B: 1k Microwire Serial EEPROM 96LC46A: 8 Bit 96LC46B: 16 Bit
IC203 = luani_chips:AP803: AP803 VCC Supervisor
IC401 IC402 = luani_chips:AP2161: 1 Channel power switch
IC501 = luani_chips:LM3671: LM3671 2MHz Step-Down
IC502 = luani_chips:74LVC2G17: Dual non-inverting schmitt buffer
IC503 = luani_chips:AP7115: 150mA LDO
J401 J402 = leo_misc-smd:JUMPER-2: Jumper
L201 L202 L502 L503 = leo_inductor-fastron:INDUCTOR: Fastron SMD Inductor
L501 = luani_inductor:L: Inductor; ARTIKEL: LQH3NPN2R2NM0L
LED201 LED301 LED401 LED402 = leo_misc-smd:LED: SMD LED
LOGO1 = leo_misc-logo:LOGO: leo-andres.de PCB Logo
MARK101-MARK104 = leo_misc-logo:FIDUCIAL: Fiducial
OSHW = leo_misc-logo:OSHW: OSHW Logo
Q201 = luani_misc-smd:CRYSTAL-SHIELD: Shielded crystal; ARTIKEL: ABM3B-25.000MHZ-B2-T
R201-R204 R302-R304 R308 R310 = leo_rc-smd:R: Resistor
R205 R402-R410 R501-R510 = luani_rc-smd:R: Resistor
R301 R305-R307 R309 R311 R401 = leo_rc-smd:R: Resistor; TOLERANZ: 1%
SP401 = leo_misc-tht:TESTPOINT: Keystone THT Testpoints (wire loop); TP_SIGNAL_NAME: +5V
SP402 = leo_misc-tht:TESTPOINT: Keystone THT Testpoints (wire loop); TP_SIGNAL_NAME: GND
SP403 = leo_misc-tht:TESTPOINT: Keystone THT Testpoints (wire loop); TP_SIGNAL_NAME: USB.DP0
SP404 = leo_misc-tht:TESTPOINT: Keystone THT Testpoints (wire loop); TP_SIGNAL_NAME: USB.DM0
T201 = leo_transistor:NPN-DIGITAL: NPN Driver/Digital (BRT) Transistor
TP1-TP8 = testpad:PTR1: TEST PIN
TVS401 = leo_diode-tvs:2-ARRAY: Dual TVS Diode Array 2 IO-Lines + VDD
TVS501 = leo_diode-tvs:TVS-UNI: TVS Diode, Unidirectional
X301 = luani_connector:MAGJACK-LED: RJ45 MagJack, 2 LEDs
X401 X402 = luani_connector:USB-4-D: Dual 4 Pin USB
X403 = luani_connector:USB-5: 5 Pin USB
X501-X503 = leo_con-pinhead:PINHD-1X1: PIN HEADER
X504 = leo_con-pinhead:PINHD-1X3: PIN HEADER
X505 = luani_connector:STEREO-JACK: Stereo jack 3 pin

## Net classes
1 USB-Diffpair: width 0.229 mm, clearance 0.508 mm to class 0, clearance 0.152 mm
2 Ethernet-Diffpair: width 0.178 mm, clearance 0.762 mm to class 0, clearance 0.762 mm to class 1, clearance 0.152 mm
3 Schirm: clearance 0.635 mm to class 0, clearance 0.635 mm to class 1, clearance 0.635 mm to class 2
4 Takt: width 0.152 mm, clearance 0.508 mm to class 0, clearance 1.27 mm to class 1, clearance 1.27 mm to class 2
5 Standardleiter neben Diffpair: clearance 0.508 mm to class 3, clearance 0.508 mm to class 4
